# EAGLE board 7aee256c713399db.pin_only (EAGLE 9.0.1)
REV: C

Size 35.56 x 17.78 mm. Coordinates in mm from the lower left corner, seen from the top.
Outline: 0,6.35 0,1.27 arc90 1.27,0 34.29,0 arc90 35.56,1.27 35.56,16.51 arc90 34.29,17.78 1.27,17.78 arc90 0,16.51 0,11.68 0.51,11.18 0.51,6.86 0,6.35
Copper layers (1*16): Top 0.035mm / dielectric 1.5mm / Bottom 0.035mm
Design rules "adafruit *": minimum track width 8mil, minimum drill 15.5mil, track to track 8mil, track to pad 8mil, pad to pad 8mil, via to via 8mil, smd to smd 8mil, copper to edge 10mil, drill to drill 8mil, minimum pad ring 10mil, minimum via ring 8mil, stop-mask expansion 2mil, vias tented up to drill 20mil, thermal gap 10mil

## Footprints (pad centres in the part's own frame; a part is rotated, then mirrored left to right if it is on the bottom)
_0603MP = smd 0.8 x 0.8: 1 -0.762,0; 2 0.762,0
0603-NO = smd 1.075 x 1: 1 -0.85,0; 2 0.85,0
0805-NO = smd 1.24 x 1.5: 1 -0.95,0; 2 0.95,0
_0805MP = smd 1.2 x 1.3: 1 -1.016,0; 2 1.016,0
SOD-123FL = smd 0.91 x 1.22: A 1.637,0; C -1.637,0
SOT23-5 = smd 0.69 x 0.99: 1 -0.95,-1.29; 2 0,-1.29; 3 0.95,-1.29; 4 0.95,1.3; 5 -0.95,1.3
TQFN48_7MM = smd 0.25 x 0.75: 1 -2.75,-3.475; 2 -2.25,-3.475; 3 -1.75,-3.475; 4 -1.25,-3.475; 5 -0.75,-3.475; 6 -0.25,-3.475; 7 0.25,-3.475; 8 0.75,-3.475; 9 1.25,-3.475; 10 1.75,-3.475; 11 2.25,-3.475; 12 2.75,-3.475; 25 2.75,3.475; 26 2.25,3.475; 27 1.75,3.475; 28 1.25,3.475; 29 0.75,3.475; 30 0.25,3.475; 31 -0.25,3.475; 32 -0.75,3.475; 33 -1.25,3.475; 34 -1.75,3.475; 35 -2.25,3.475; 36 -2.75,3.475 | smd 0.75 x 0.25: 13 3.475,-2.75; 14 3.475,-2.25; 15 3.475,-1.75; 16 3.475,-1.25; 17 3.475,-0.75; 18 3.475,-0.25; 19 3.475,0.25; 20 3.475,0.75; 21 3.475,1.25; 22 3.475,1.75; 23 3.475,2.25; 24 3.475,2.75; 37 -3.475,2.75; 38 -3.475,2.25; 39 -3.475,1.75; 40 -3.475,1.25; 41 -3.475,0.75; 42 -3.475,0.25; 43 -3.475,-0.25; 44 -3.475,-0.75; 45 -3.475,-1.25; 46 -3.475,-1.75; 47 -3.475,-2.25; 48 -3.475,-2.75 | smd 4.7 x 4.7: THERMAL 0,0
1X05_ROUND_70 = drill 1 pad 1.778: 1 -5.08,0; 2 -2.54,0; 3 0,0; 4 2.54,0; 5 5.08,0
1X14_ROUND70 = drill 1 pad 1.676: 1 -16.51,0; 2 -13.97,0; 3 -11.43,0; 4 -8.89,0; 5 -6.35,0; 6 -3.81,0; 7 -1.27,0; 8 1.27,0; 9 3.81,0; 10 6.35,0; 11 8.89,0; 12 11.43,0; 13 13.97,0; 14 16.51,0
CHIPLED_0603_NOOUTLINE = smd 0.8 x 0.8: A 0,-0.75; C 0,0.75
APA102_2020 = smd 0.7 x 0.35: 1 -0.95,-0.75; 2 -0.95,0; 3 -0.95,0.75; 4 0.95,0.75; 5 0.95,0; 6 0.95,-0.75
SOLDERJUMPER_CLOSEDWIRE = smd 1.168 x 1.6: 1 -0.762,0; 2 0.762,0 | smd 0.635 x 0.203: WIRE 0,0
KMR2 = smd 1 x 1: 1 2,0.8; 2 2,-0.8; 3 -2,0.8; 4 -2,-0.8
USON8 = smd 0.35 x 0.25: 1 -1.2,0.75; 2 -1.2,0.25; 3 -1.2,-0.25; 4 -1.2,-0.75; 5 1.2,-0.75; 6 1.2,-0.25; 7 1.2,0.25; 8 1.2,0.75
SOT23-5' = smd 0.55 x 1.2: 1 -0.95,-1.3; 2 0,-1.3; 3 0.95,-1.3; 4 0.95,1.3; 5 -0.95,1.3
FIDUCIAL_1MM = smd 1 x 1: 1 0,0
4UCONN_20329_V2 = smd 1 x 2: BASE@1 -0.75,-2; BASE@2 0.75,-2 | smd 0.4 x 1.35: D+ 0,0.775; D- -0.65,0.775; GND 1.3,0.775; ID 0.65,0.775; VBUS -1.3,0.775 | drill 0.8 pad 1.143 offset: SPRT@1 -3.3,0.9; SPRT@2 3.3,0.9 | drill 0.9 pad 2.413 square: SPRT@3 -3.6,-1.9; SPRT@4 3.6,-1.9 | hole 0.7: -1.95,0; 1.95,0

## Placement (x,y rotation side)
C1  1uF  [_0603MP]  30.48,5.91 0 top
C5  1uF  [0603-NO]  28.32,8.32 90 top
C6  10µF  [0805-NO]  12.58,13.38 0 top
C7  1uF  [0603-NO]  11.45,10.78 90 top
C8  10µF  [0805-NO]  8.45,4.18 180 top
C9  10uF  [_0805MP]  13.27,10.22 90 top
C14  1uF  [0603-NO]  6.77,7.16 90 top
D1  MBR120  [SOD-123FL]  8.57,13.46 180 top
D2  MBR120  [SOD-123FL]  8.57,11.68 180 top
IC1  74HCT1G125DBV  [SOT23-5]  24.07,13.08 90 top
IC2  ATSAMD51G_TQFN48  [TQFN48_7MM]  19.18,7.94 0 top
JP1  [1X05_ROUND_70]  34.29,8.89 90 top
JP2  [1X14_ROUND70]  17.78,16.51 0 top
JP4  [1X14_ROUND70]  17.78,1.27 180 top
L  RED  [CHIPLED_0603_NOOUTLINE]  31.54,13.38 180 top
L2  AP102-2020  [APA102_2020]  12.06,4.83 0 top
R1  100k  [0603-NO]  9.14,10.03 180 top
R2  100k  [0603-NO]  26.04,9.21 180 top
R3  2.2K  [_0603MP]  30.48,4.89 180 top
R4  10K  [_0603MP]  29.02,3.87 0 top
R7  2.2K  [0603-NO]  29.21,13.78 0 top
SJ1  [SOLDERJUMPER_CLOSEDWIRE]  7.62,4.51 90 bottom
SW1  SPST_TACT-KMR2  [KMR2]  30.48,9.02 270 top
U1  GD25x16  [USON8]  26.29,5.14 270 top
U2  AP2112K-3.3  [SOT23-5']  9.27,7.24 180 top
U$4  [ITSYM4_TOP]  0,0 0 top
U$5  [ITSYM4_BOT]  35.56,0 0 bottom
U$6  [PCBFEAT-REV-040]  12.13,7.49 0 top
U$34  FIDUCIAL_1MM  [FIDUCIAL_1MM]  30.23,9.4 270 top
U$35  FIDUCIAL_1MM  [FIDUCIAL_1MM]  2.21,3.06 270 top
X3  microUSB  [4UCONN_20329_V2]  4.45,8.89 270 top

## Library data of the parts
C1 C5-C7 C9 C14 IC2 JP1 JP2 JP4 L L2 R1-R4 R7 SJ1 U1 U2 U$6 X3 = microbuilder
C8 = microbuilder; COMPANY: ADAFRUIT INDUSTRIES; DRAWN: KTOWN; REV: A
D1 D2 SW1 = adafruit
IC1 = 74xx-little-us
U$4 U$5 = silks
U$34 U$35 = microbuilder; BOM: EXCLUDE

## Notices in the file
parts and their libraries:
microbuilder: This work is placed in the public domain, and may be freely used for commercial and non-commercial work with the following conditions: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
